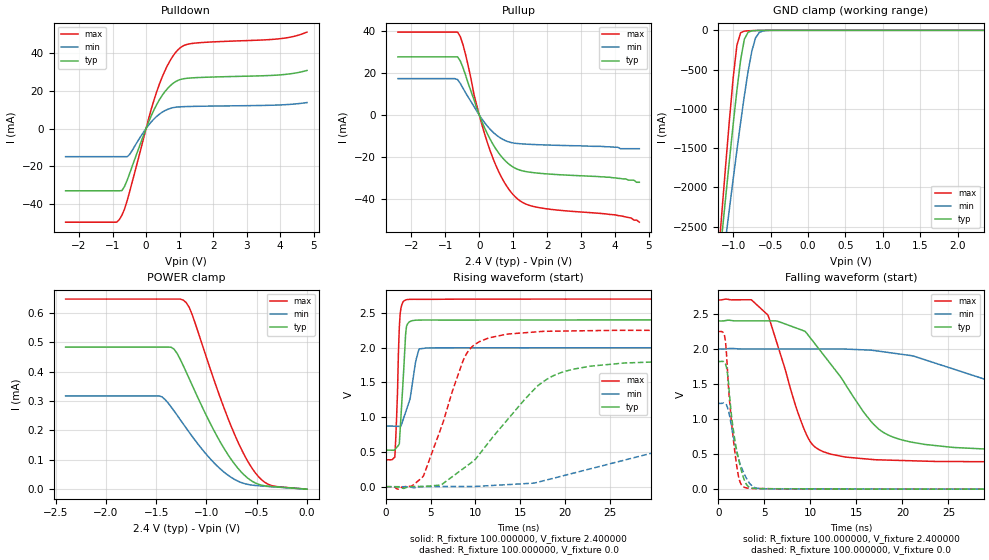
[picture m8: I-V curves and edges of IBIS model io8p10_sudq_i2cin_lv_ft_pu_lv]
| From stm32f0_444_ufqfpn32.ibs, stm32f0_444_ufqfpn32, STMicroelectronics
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|   Model io8p10_sudq_i2cin_lv_ft_pu_lv
[Model]  io8p10_sudq_i2cin_lv_ft_pu_lv
Model_type I/O
Polarity   Non-Inverting
Enable   Active-Low
Vinl =   0.720000V
Vinh =   1.680000V
Vmeas =  1.200000V
Cref =   50.000000pF
Rref =   100.000000M
Vref =   0.0V
C_comp   2.067900pF   1.988600pF   2.164800pF
[Temperature Range]   25.000000   0.125000k   -40.000000
[Pullup Reference]   2.400000V   2.000000V   2.700000V
[Pulldown Reference]   0.0V   0.0V   0.0V
[POWER Clamp Reference]   2.400000V   2.000000V   2.700000V
[GND Clamp Reference]   0.0V   0.0V   0.0V
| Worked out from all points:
|   slope of the pulldown table from 0 to 0.36 V, typ, clamps not added: 25.5 ohm
|   slope of the pullup table from 0 to 0.36 V, typ, clamps not added: 28.4 ohm
|   GND clamp passes 1 mA (typ) near -0.64 V on its own axis
|   rising waveform, R_fixture 100.000000, V_fixture 2.400000: 20-80 % time 501ps typ, 1.02ns min, 334ps max; typ from 0.527 V to 2.4 V
|   rising waveform, R_fixture 100.000000, V_fixture 0.0: 20-80 % time 7.27ns typ, 22.1ns min, 3.54ns max; typ from 0.001 V to 1.82 V
|   falling waveform, R_fixture 100.000000, V_fixture 2.400000: 20-80 % time 6.28ns typ, 18.8ns min, 3.34ns max; typ from 2.4 V to 0.527 V
|   falling waveform, R_fixture 100.000000, V_fixture 0.0: 20-80 % time 1.17ns typ, 1.4ns min, 928ps max; typ from 1.82 V to 0.001 V
[Pulldown]
|Voltage   I(typ)   I(min)   I(max)
-2.4V     -33.16mA   -14.98mA   -49.86mA
-880mV    -33.16mA   -14.98mA   -49.86mA
-800mV    -33.16mA   -14.98mA   -48.55mA
-640mV    -30.75mA   -14.98mA   -42.77mA
-480mV    -23.43mA   -13.57mA   -32.92mA
80mV      3.651mA    1.905mA    5.506mA
400mV     15.37mA    7.665mA    23.73mA
720mV     22.75mA    10.69mA    36.23mA
1.04V     26.18mA    11.57mA    43.27mA
1.52V     27.09mA    11.81mA    45.55mA
4V        28.55mA    12.55mA    47.81mA
4.8V      30.9mA     13.81mA    51.31mA
[Pullup]
|Voltage   I(typ)   I(min)   I(max)
-2.4V     27.74mA    17.36mA    39.51mA
-640mV    27.74mA    16.89mA    39.51mA
-560mV    25.73mA    15.05mA    37.34mA
-480mV    22.59mA    12.74mA    33.43mA
-80mV     3.427mA    2.072mA    4.957mA
160mV     -6.219mA   -3.714mA   -9.136mA
320mV     -11.51mA   -6.781mA   -16.98mA
720mV     -21mA      -11.8mA    -31.53mA
1.12V     -25.77mA   -13.54mA   -39.82mA
1.76V     -27.69mA   -14.12mA   -44.06mA
4V        -29.9mA    -15.3mA    -47.5mA
4.72V     -32mA      -16mA      -51mA
[GND_clamp]
|Voltage   I(typ)   I(min)   I(max)
-2.4V     -9.567A    -9.921A    -9.731A
-1.2V     -3.09A     -3.428A    -2.911A
-1.15V    -2.606A    -3.04A     -2.31A
-1.1V     -2.127A    -2.655A    -1.719A
-1.05V    -1.657A    -2.274A    -1.146A
-950mV    -765.3mA   -1.53A     -190.2mA
-900mV    -376.6mA   -1.172A    -30.81mA
-850mV    -112.3mA   -832.5mA   -10.23mA
-750mV    -6.57mA    -264.6mA   -4.026mA
-700mV    -2.581mA   -94.26mA   -2.329mA
-600mV    -416.4uA   -8.158mA   -368uA
2.35V     0A         0A         0A
[POWER_clamp]
|Voltage   I(typ)   I(min)   I(max)
-2.4V     483.6uA    317.3uA    647uA
-1.47V    483.6uA    317.3uA    647uA
-1.32V    475.8uA    265.5uA    647uA
-1.23V    420.2uA    221.8uA    643.4uA
-1.17V    375.2uA    193uA      618uA
-1.14V    352.5uA    178.9uA    592.4uA
-840mV    147.3uA    62.31uA    290.1uA
-690mV    72.45uA    27.82uA    163.1uA
-540mV    25.82uA    13.54uA    67.87uA
-450mV    13.39uA    10.73uA    31.49uA
-360mV    9.214uA    8.518uA    13uA
0V        0A         0A         0A
[Ramp]
| variable   typ   min   max
dV/dt_r  1.09275/7.26473n   0.73293/22.08271n   1.34920/3.54056n
dV/dt_f  1.12393/6.27325n   0.67486/18.80501n   1.38687/3.33248n
R_load = 100.000000
[Rising Waveform]
R_fixture= 100.000000
V_fixture= 2.400000
V_fixture_min= 2.000000
V_fixture_max= 2.700000
|time   V(typ)   V(min)   V(max)
0s        526.5mV    872.5mV    388.6mV
1.001ns   534.5mV    870.8mV    427.8mV
1.301ns   580mV      869.3mV    1.368V
1.401ns   595.2mV    869mV      1.925V
1.502ns   617.7mV    868.7mV    2.296V
1.702ns   1.048V     879mV      2.581V
2.202ns   2.19V      1.072V     2.687V
2.503ns   2.356V     1.187V     2.695V
3.704ns   2.398V     1.983V     2.696V
49.85ns   2.4V       2V         2.7V
[Rising Waveform]
R_fixture= 100.000000
V_fixture= 0.0
V_fixture_min= 0.0
V_fixture_max= 0.0
|time   V(typ)   V(min)   V(max)
0s        1.055mV    1.354mV    939.9uV
2.803ns   2.595mV    -5.333mV   6.013mV
4.204ns   4.255mV    3.374mV    158.2mV
6.206ns   29.86mV    4.223mV    863.5mV
9.009ns   297.7mV    4.563mV    1.915V
13.41ns   941.4mV    29.97mV    2.193V
18.62ns   1.593V     120.3mV    2.238V
26.63ns   1.781V     383.8mV    2.25V
51.45ns   1.823V     1.103V     2.25V
99.7ns    1.822V     1.224V     2.25V
[Falling Waveform]
R_fixture= 100.000000
V_fixture= 2.400000
V_fixture_min= 2.000000
V_fixture_max= 2.700000
|time   V(typ)   V(min)   V(max)
0s        2.4V       2V         2.7V
3.604ns   2.401V     2V         2.702V
5.405ns   2.402V     2V         2.484V
9.81ns    2.192V     2V         719.2mV
13.81ns   1.495V     1.999V     458.7mV
18.02ns   804.4mV    1.959V     417mV
25.43ns   597.3mV    1.719V     395.2mV
34.43ns   550.7mV    1.333V     389.1mV
50.25ns   530.2mV    964.3mV    388.5mV
99.7ns    526.5mV    872.5mV    388.6mV
[Falling Waveform]
R_fixture= 100.000000
V_fixture= 0.0
V_fixture_min= 0.0
V_fixture_max= 0.0
|time   V(typ)   V(min)   V(max)
0s        1.822V     1.224V     2.25V
700.7ps   1.803V     1.224V     2.181V
1.001ns   1.658V     1.167V     1.713V
1.401ns   1.1V       928.1mV    1.015V
1.902ns   627.7mV    599.2mV    437.8mV
2.302ns   380mV      395.2mV    130.8mV
2.903ns   110mV      197.7mV    24.56mV
3.704ns   16.12mV    43.53mV    10.89mV
4.905ns   7.831mV    7.576mV    9.452mV
49.85ns   1.055mV    1.354mV    939.9uV
